(* Logix 5000 DataType export DriveFaults; software revision 20.01 *)

TYPE DriveFaults :
STRUCT
   Positive_Limit : BOOL;   // Positive Limit
   Negative_Limit : BOOL;   // Negative Limit
   E_Stop : BOOL;   // E Stop
   Position_Error : BOOL;   // Position Error
   Feedback_Error : BOOL;   // Feedback Error
   Over_Current : BOOL;   // Overcurrent
   Motor_Over_Temperature : BOOL;   // Motor Over Temperature
   Drive_Over_Temperature : BOOL;   // Drive Over Temperature
   Drive_Over_Voltage : BOOL;   // Drive Over Voltage
   Drive_Under_Voltage : BOOL;   // Drive Under Voltage
   Flash_Error : BOOL;   // Flash Error
   I2T_Limit : BOOL;   // I2T Limit Fault
   Short_Circuit : BOOL;   // Short Circuit Fault
   Watchdog_Reset : BOOL;   // Watchdog Reset
END_STRUCT
END_TYPE
